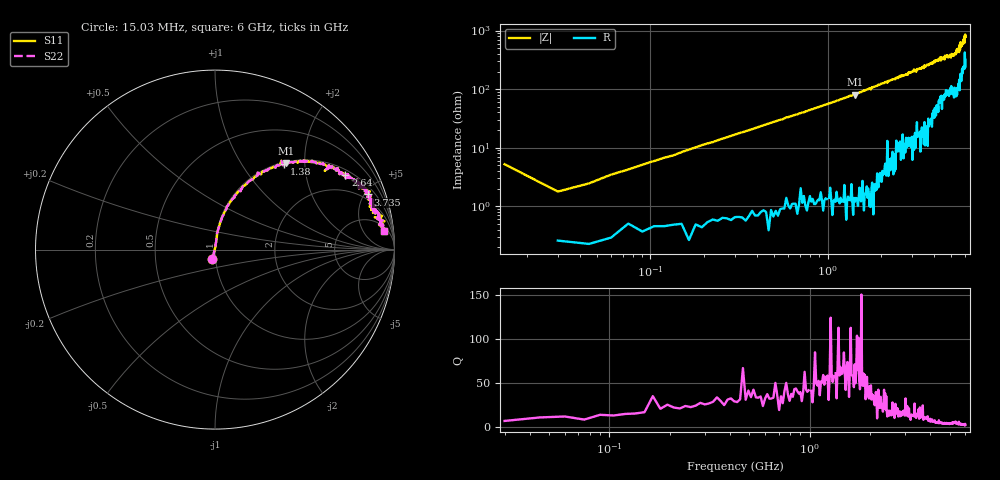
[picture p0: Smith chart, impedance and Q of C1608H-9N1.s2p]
!	Network	Analyzer	HP8753E.07.74:	Oct	30	2002	Serial	No.	JP38451487
!	Hewlett-Packard
!	7	Sep	2009	10:16:10
!	Frequency	S11	S21	S12	S22
#	HZ	S	RI	R	50
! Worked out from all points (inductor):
!   400 points, 15.03 MHz to 6 GHz, reference 50 ohm
!   read as one part in series: L = 8.93 nH near 45.03 MHz
!   highest Q = 67.1 at 1.425 GHz (marker M1), where L = 9.03 nH
!   S11 on the Smith chart (normalised r, x): 15.03 MHz: 0.97, -0.10; 1.38 GHz: 1.02, +1.57; 2.64 GHz: 1.21, +3.36; 3.735 GHz: 1.57, +5.26; 6 GHz: 7, +14
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1.502992e7  -0.0145 -0.0514  1.01 0.0514  1.01 0.0514  -0.0145 -0.0514
3.002985e7  0.00277 0.0175  0.997 -0.0175  0.997 -0.0175  0.00277 0.0175
6.00297e7  0.00417 0.0343  0.996 -0.0343  0.996 -0.0343  0.00417 0.0343
1.200294e8  0.00899 0.0664  0.991 -0.0664  0.991 -0.0664  0.00899 0.0664
2.850286e8  0.0298 0.153  0.97 -0.153  0.97 -0.153  0.0298 0.153
5.850271e8  0.108 0.29  0.892 -0.29  0.892 -0.29  0.108 0.29
1.020025e9  0.25 0.421  0.75 -0.421  0.75 -0.421  0.25 0.421
1.380023e9  0.384 0.479  0.616 -0.479  0.616 -0.479  0.384 0.479
1.425023e9  0.397 0.482  0.603 -0.482  0.603 -0.482  0.397 0.482
2.01002e9  0.598 0.476  0.402 -0.476  0.402 -0.476  0.598 0.476
2.640017e9  0.727 0.415  0.273 -0.415  0.273 -0.415  0.727 0.415
3.015015e9  0.793 0.39  0.207 -0.39  0.207 -0.39  0.793 0.39
3.735011e9  0.85 0.307  0.15 -0.307  0.15 -0.307  0.85 0.307
4.00501e9  0.878 0.278  0.122 -0.278  0.122 -0.278  0.878 0.278
5.010005e9  0.884 0.215  0.116 -0.215  0.116 -0.215  0.884 0.215
5.535002e9  0.89 0.181  0.11 -0.181  0.11 -0.181  0.89 0.181
5.625002e9  0.937 0.136  0.0634 -0.136  0.0634 -0.136  0.937 0.136
5.655002e9  0.92 0.159  0.0798 -0.159  0.0798 -0.159  0.92 0.159
5.865001e9  0.941 0.12  0.0587 -0.12  0.0587 -0.12  0.941 0.12
5.925e9  0.925 0.133  0.0749 -0.133  0.0749 -0.133  0.925 0.133
5.955e9  0.933 0.0913  0.0673 -0.0913  0.0673 -0.0913  0.933 0.0913
6e9  0.94 0.104  0.0601 -0.104  0.0601 -0.104  0.94 0.104
